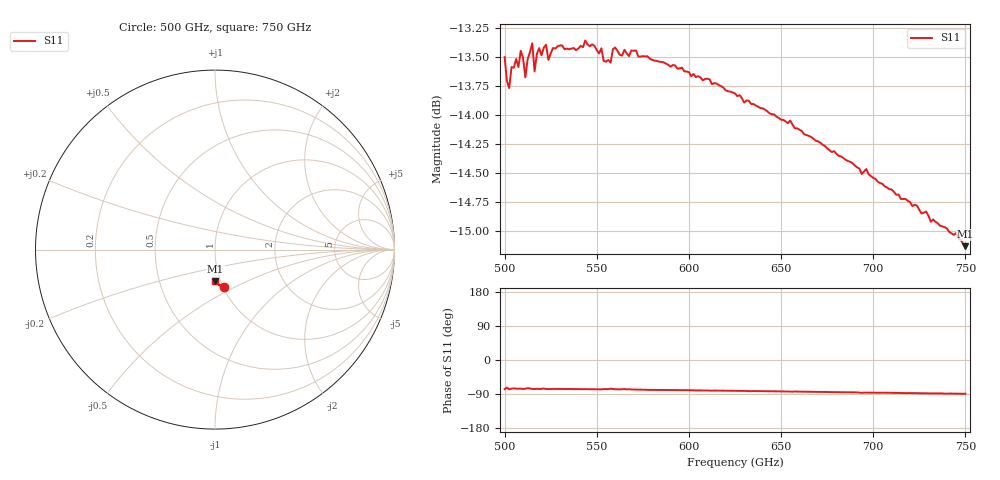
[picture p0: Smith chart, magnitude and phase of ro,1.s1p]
!Created with mwavepy.
!Created with skrf (http://scikit-rf.org).
# GHz S RI R 50.0
!freq ReS11 ImS11
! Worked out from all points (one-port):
!   201 points, 500 GHz to 750 GHz, reference 50 ohm
!   lowest |S11| = -15.1 dB at 750 GHz (marker M1), VSWR 1.42, Z = 47.3 - j17.1 ohm
!   |S11| at or under -10 dB: start of sweep to end of sweep
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500  0.0477 -0.2059
501.25  0.0613 -0.1971
502.5  0.0443 -0.2001
503.75  0.0523 -0.2026
505  0.0549 -0.2018
507.5  0.0512 -0.2029
508.75  0.0529 -0.206
511.25  0.0508 -0.2008
512.5  0.0572 -0.203
515  0.0514 -0.208
516.25  0.0481 -0.2027
518.75  0.0499 -0.2073
521.25  0.0548 -0.2062
522.5  0.0497 -0.2081
523.75  0.0489 -0.205
531.25  0.0499 -0.2079
543.75  0.0494 -0.2091
552.5  0.0462 -0.2081
553.75  0.0483 -0.2049
557.5  0.0519 -0.2037
558.75  0.0503 -0.207
562.5  0.0461 -0.2067
593.75  0.0382 -0.2054
625  0.0302 -0.2016
656.25  0.0221 -0.1963
687.5  0.0162 -0.1897
718.75  0.0083 -0.183
750  0.0025 -0.1751
